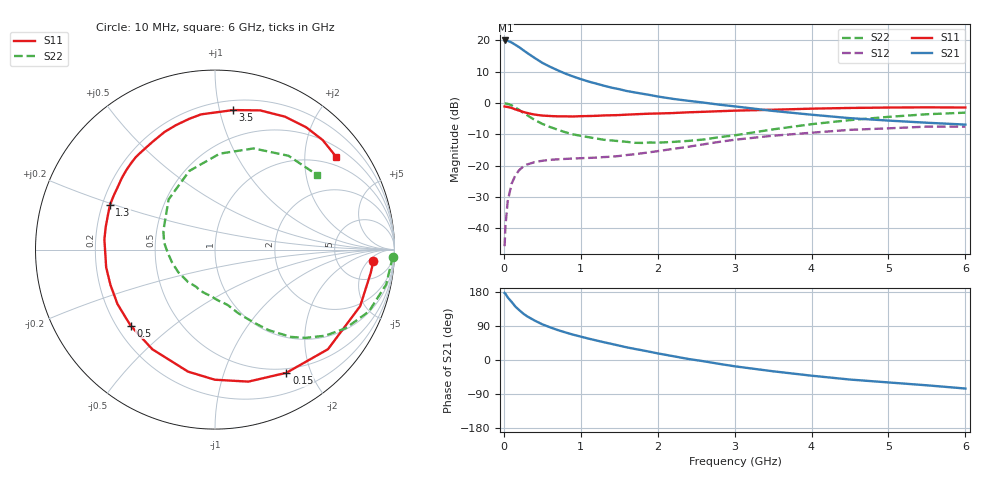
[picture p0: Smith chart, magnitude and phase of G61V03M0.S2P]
! SIEMENS Small Signal Semiconductors
! BFG193
! Si NPN RF Bipolar Junction Transistor in SOT223
! VCE = 1 V  IC = 3 mA
! Common Emitter S-Parameters:  August  1996
# GHz  S  MA  R  50
!  f  S11  S21  S12  S22
! GHz  MAG  ANG  MAG  ANG  MAG  ANG  MAG  ANG
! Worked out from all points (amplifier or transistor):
!   36 points, 10 MHz to 6 GHz, reference 50 ohm
!   highest |S21| = 20.0 dB at 20 MHz (marker M1)
!   |S21| within 3 dB of that: start of sweep to 246.5 MHz
!   unconditionally stable (mu >= 1): 1.234 GHz to 2.94 GHz
!   at 250 MHz: K = 0.24, MSG = 18.6 dB, |S12| = -20.3 dB
!   at 1.4 GHz: K = 1.09, MAG = 9.2 dB, |S12| = -17.1 dB
!   at 6 GHz: K = 0.99, MSG = 0.3 dB, |S12| = -7.5 dB
!   S11 on the Smith chart (normalised r, x): 10 MHz: 12, -7; 150 MHz: 0.44, -1.65; 500 MHz: 0.26, -0.36; 1.3 GHz: 0.23, +0.19; 3.5 GHz: 0.27, +1.10; 6 GHz: 0.74, +2.77
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0.01  0.8841 -4.3  9.965 177.0  0.0052 89.1  0.9912 -2.3
0.02  0.8773 -8.5  10.01 175.2  0.0106 85.8  0.9843 -4.6
0.05  0.868 -21.3  9.859 165.3  0.027 78.5  0.9735 -11.5
0.1  0.8392 -41.4  9.295 153.7  0.0513 68.5  0.9243 -21.9
0.15  0.7933 -59.9  8.525 140.9  0.0704 58.3  0.8492 -31.1
0.2  0.7587 -75.8  7.801 131.7  0.0852 51.5  0.7792 -38.0
0.25  0.725 -90.1  7.033 122.8  0.0967 45.1  0.7041 -44.3
0.3  0.6962 -102.5  6.367 115.6  0.1044 40.3  0.6447 -49.0
0.4  0.6558 -122.2  5.266 104.2  0.1142 33.2  0.5395 -56.3
0.5  0.6328 -138.0  4.397 94.2  0.1201 28.0  0.4662 -61.5
0.6  0.6223 -150.8  3.81 86.3  0.1242 25.1  0.4158 -65.8
0.7  0.6149 -161.3  3.343 79.1  0.1266 23.0  0.3764 -70.0
0.9  0.6116 -177.9  2.662 66.9  0.1304 20.8  0.3172 -77.0
1.1  0.6218 168.4  2.213 56.5  0.1333 20.1  0.2859 -85.8
1.3  0.6358 157.1  1.898 46.9  0.1376 20.6  0.2597 -94.5
1.6  0.6545 142.5  1.558 33.3  0.1483 21.6  0.2407 -111.1
2.2  0.694 120.1  1.168 10.1  0.1858 21.3  0.2402 -148.5
2.8  0.7425 101.2  0.944 -10.2  0.2405 14.9  0.2858 172.4
3.5  0.7839 82.6  0.75 -29.8  0.3016 0.6  0.3807 132.8
4.5  0.8368 62.3  0.575 -51.6  0.3744 -19.6  0.5352 87.2
5.5  0.8558 45.5  0.486 -66.8  0.4215 -44.3  0.6641 51.9
6  0.8503 37.5  0.454 -75.3  0.4219 -58.1  0.7042 36.3
